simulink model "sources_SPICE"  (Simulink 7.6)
settings: Solver=ode15s  StartTime=0.0  StopTime=10.0  RelTol=1e-3
StopFcn:
  | close all
  | load signaux.mat
  | plot(x(1,:),x(2,:))
  | axis([0 10 -1 6])
  | grid
  | title('Courant dans la résistance R')
  | xlabel('temps')
libraries: fl_lib x7, nesl_utility x4, elec_lib x3

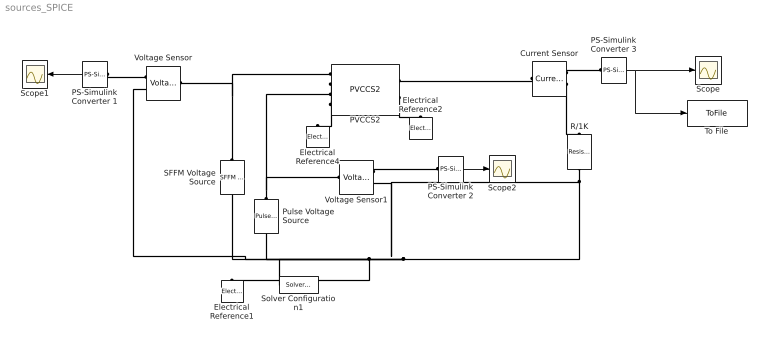
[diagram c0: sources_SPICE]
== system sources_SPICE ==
  Current Sensor : fl_lib/Electrical/Electrical Sensors/Current Sensor  DialogController=NetworkEngine.DynNeDlgSource  SystemSampleTime=-1  i1_Log=off  v1_Log=off  LocalVarNames=|i1|v1  LocalVarDescs=|i1|v1  LocalVarLogging=[0 0]
  Electrical Reference1 : fl_lib/Electrical/Electrical Elements/Electrical Reference  DialogController=NetworkEngine.DynNeDlgSource  SystemSampleTime=-1  i_Log=off  LocalVarNames=|i  LocalVarDescs=|i  LocalVarLogging=[]
  Electrical Reference2 : fl_lib/Electrical/Electrical Elements/Electrical Reference  DialogController=NetworkEngine.DynNeDlgSource  SystemSampleTime=-1  i_Log=off  LocalVarNames=|i  LocalVarDescs=|i  LocalVarLogging=[]
  Electrical Reference4 : fl_lib/Electrical/Electrical Elements/Electrical Reference  DialogController=NetworkEngine.DynNeDlgSource  SystemSampleTime=-1  i_Log=off  LocalVarNames=|i  LocalVarDescs=|i  LocalVarLogging=[]
  PS-Simulink Converter 1 : nesl_utility/PS-Simulink Converter  DialogController=NetworkEngine.DynNeUtilDlgSource  SystemSampleTime=-1  PhysicalDomain=network_engine_domain  LeftPortType=input  RightPortType=output  SubClassName=ps_output  Unit=1  AffineConversion=off
  PS-Simulink Converter 2 : nesl_utility/PS-Simulink Converter  DialogController=NetworkEngine.DynNeUtilDlgSource  SystemSampleTime=-1  PhysicalDomain=network_engine_domain  LeftPortType=input  RightPortType=output  SubClassName=ps_output  Unit=1  AffineConversion=off
  PS-Simulink Converter 3 : nesl_utility/PS-Simulink Converter  DialogController=NetworkEngine.DynNeUtilDlgSource  SystemSampleTime=-1  PhysicalDomain=network_engine_domain  LeftPortType=input  RightPortType=output  SubClassName=ps_output  Unit=1  AffineConversion=off
  PVCCS2 : elec_lib/Additional Components/SPICE-Compatible Components/Sources/PVCCS2  DialogController=NetworkEngine.DynNeDlgSource  SystemSampleTime=-1  PEES=[0 0.5 1]  LocalVarLogging=[]
  Pulse Voltage Source : elec_lib/Additional Components/SPICE-Compatible Components/Sources/Pulse Voltage Source  DialogController=NetworkEngine.DynNeDlgSource  SystemSampleTime=-1  V1=0 V  V2=5 V  TD=0 s  TR=1e-09 s  TF=1e-09 s  PW=2 s  PER=4 s  voltage_Log=off  LocalVarNames=|voltage  LocalVarDescs=|Voltage (V)  LocalVarLogging=0
  R/1K : fl_lib/Electrical/Electrical Elements/Resistor  DialogController=NetworkEngine.DynNeDlgSource  SystemSampleTime=-1  R=1 kOhm  i_Log=off  v_Log=off  LocalVarNames=|i|v  LocalVarDescs=|i|v  LocalVarLogging=[0 0]
  SFFM Voltage Source : elec_lib/Additional Components/SPICE-Compatible Components/Sources/SFFM Voltage Source  DialogController=NetworkEngine.DynNeDlgSource  SystemSampleTime=-1  VO=0 V  VA=1 V  FC=0.5 Hz  MI=0  FS=0 Hz  current_Log=off  voltage_Log=off  power_Log=off  LocalVarNames=|current|voltage|power  LocalVarDescs=|Current (A)|Voltage (V)|Power (W)  LocalVarLogging=[0 0 0]
  Scope : Scope
  Scope1 : Scope
  Scope2 : Scope
  Solver Configuration1 : nesl_utility/Solver Configuration  DialogController=NetworkEngine.DynNeUtilDlgSource  SystemSampleTime=-1  PhysicalDomain=network_engine_domain  LeftPortType=input  RightPortType=generic  SubClassName=solver  Accelerate=off  Profile=off  ResidualTolerance=1e-9  MaxNonlinIter=12  MaxModeIter=2  DoFixedCost=off  UseLocalSampling=off  DoDC=off  LinearAlgebra=Sparse  LocalSolverSampleTime=.001  LocalSolverChoice=NE_BACKWARD_EULER_ADVANCER  UseLocalSolver=off
  To File : ToFile  Filename=signaux  MatrixName=x
  Voltage Sensor : fl_lib/Electrical/Electrical Sensors/Voltage Sensor  DialogController=NetworkEngine.DynNeDlgSource  SystemSampleTime=-1  i1_Log=off  v1_Log=off  LocalVarNames=|i1|v1  LocalVarDescs=|i1|v1  LocalVarLogging=[0 0]
  Voltage Sensor1 : fl_lib/Electrical/Electrical Sensors/Voltage Sensor  DialogController=NetworkEngine.DynNeDlgSource  SystemSampleTime=-1  i1_Log=off  v1_Log=off  LocalVarNames=|i1|v1  LocalVarDescs=|i1|v1  LocalVarLogging=[0 0]
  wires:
  PS-Simulink Converter 3/1 -> Scope/1, To File/1
  PS-Simulink Converter 1/1 -> Scope1/1
  PS-Simulink Converter 2/1 -> Scope2/1
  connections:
  Pulse Voltage Source/LConn1 -- PVCCS2/LConn3 -- Voltage Sensor1/LConn1
  SFFM Voltage Source/LConn1 -- PVCCS2/LConn1 -- Voltage Sensor/LConn1
  PVCCS2/LConn4 -- PVCCS2/LConn2 -- Electrical Reference4/LConn1
  Current Sensor/LConn1 -- PVCCS2/RConn1
  Current Sensor/RConn1 -- PS-Simulink Converter 3/LConn1
  R/1K/LConn1 -- Solver Configuration1/RConn1 -- SFFM Voltage Source/RConn1 -- Electrical Reference1/LConn1 -- Voltage Sensor/RConn2 -- Pulse Voltage Source/RConn1 -- Voltage Sensor1/RConn2
  Current Sensor/RConn2 -- R/1K/RConn1
  PS-Simulink Converter 1/LConn1 -- Voltage Sensor/RConn1
  Voltage Sensor1/RConn1 -- PS-Simulink Converter 2/LConn1
  PVCCS2/RConn2 -- Electrical Reference2/LConn1
